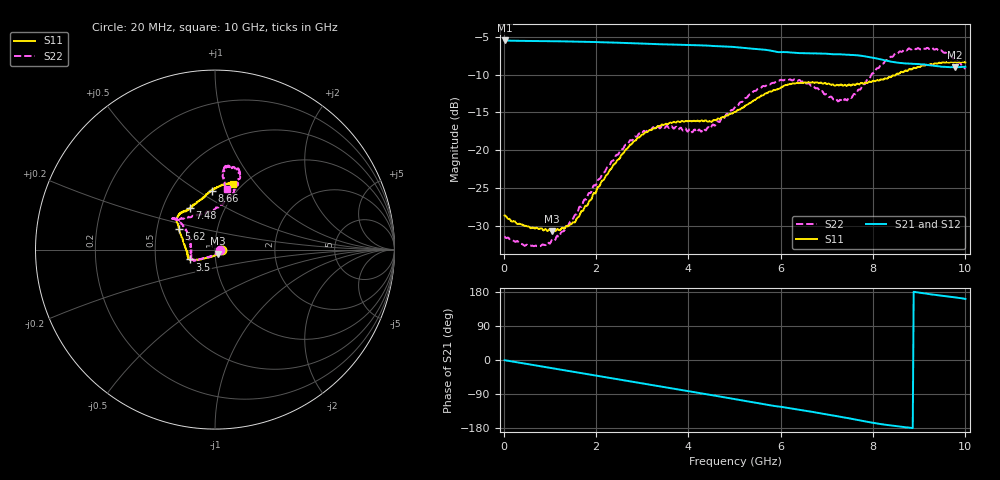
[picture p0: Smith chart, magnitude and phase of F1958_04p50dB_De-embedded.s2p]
! Integrated Device Technology
! Corporate Headquarters
! 6024 Silver Creek Valley Road
! San Jose, CA 95138  USA
! Phone:  1-408-284-8200
! Toll Free:  1-800-223-1366
! Webpage:  http://www.idt.com/
! Timing and RF Division
! 515 Groton Road, Suite 102
! Westford, MA 01886-6024
! Device:  F1958
! Description: 7-bit 0.25 dB Digital Step Attenuator
! Frequency:  0.001 -  6.000 GHz
! Package:  4x4 mm Thin QFN Plastic Package: 24 pin
! Ports:  2 RF, 12 DC
!  Pin  1  = D0
!  Pin  2  = VDD
!  Pin  3  = VMODE
!  Pin  4  = GND
!  Pin  5  = RF1  =  Port 1
!  Pin  6  = GND
!  Pin  7  = GND
!  Pin  8  = GND
!  Pin  9  = GND
!  Pin 10  = GND
!  Pin 11  = GND
!  Pin 12  = GND
!  Pin 13  = GND
!  Pin 14  = RF2  =  Port 2
!  Pin 15  = GND
!  Pin 16  = LE
!  Pin 17  = CLK
!  Pin 18  = DATA
!  Pin 19  = D6
!  Pin 20  = D5
!  Pin 21  = D4
!  Pin 22  = D3
!  Pin 23  = D2
!  Pin 24  = D1
! State:  18
! Atten State:  4.50 dB
! Voltage:  +3.30 Volts
! Current:  0.258 mA
! Data:  The device was measured on a F1958 evaluation board which has
!  individual transmission lines to the RF pins.  Data was collected
!  using a calibrated network analyzer.  The evaluation board was
!  de-embedded using Automatic Fixture Removal (AFR).
!  The reference plane is the edge of the package pin.
! Misc:
!  Action Tracker AT0419
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# GHz S dB R 50
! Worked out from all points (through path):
!   500 points, 20 MHz to 10 GHz, reference 50 ohm
!   highest |S21| = -5.51 dB at 20 MHz (marker M1); lowest = -9.0 dB at 9.78 GHz (marker M2)
!   group delay of S21, straight-line fit = 56.3 ps
!   lowest |S11| = -30.7 dB at 1.04 GHz (marker M3), VSWR 1.06, Z = 51.8 - j2.38 ohm
!   |S11| at or under -10 dB: start of sweep to 8.497 GHz
!   |S22| runs from -32.6 to -6.5 dB; largest |S21 - S12| = 0.0017
!   S11 on the Smith chart (normalised r, x): 20 MHz: 1.08, -0.00; 3.5 GHz: 0.75, -0.08; 5.62 GHz: 0.65, +0.16; 7.48 GHz: 0.68, +0.34; 8.66 GHz: 0.78, +0.57; 10 GHz: 0.91, +0.78
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0.02  -28.60 -3.4  -5.51 -0.6  -5.51 -0.5  -31.36 -4.3
0.56  -30.14 -21.0  -5.57 -11.6  -5.57 -11.6  -32.58 -29.7
1.04  -30.68 -51.6  -5.60 -21.4  -5.60 -21.4  -31.84 -69.3
1.42  -29.89 -86.6  -5.64 -29.3  -5.64 -29.3  -29.62 -104.0
1.7  -28.00 -107.4  -5.68 -34.9  -5.67 -34.9  -27.27 -122.2
2.6  -20.32 -145.9  -5.83 -53.5  -5.82 -53.5  -19.67 -148.8
2.96  -18.17 -152.6  -5.91 -61.0  -5.90 -61.0  -17.82 -151.4
3.36  -16.83 -156.6  -6.00 -69.1  -6.00 -69.2  -16.98 -155.4
3.5  -16.52 -158.6  -6.02 -72.0  -6.03 -72.1  -16.99 -159.3
4.32  -16.16 -170.8  -6.16 -88.9  -6.18 -88.9  -17.17 173.2
5.02  -14.94 166.9  -6.38 -103.6  -6.39 -103.6  -14.19 146.5
5.62  -12.74 150.4  -6.71 -116.2  -6.72 -116.2  -11.50 141.6
6.18  -11.27 141.6  -7.08 -126.9  -7.09 -126.9  -10.69 143.2
6.68  -11.02 134.4  -7.21 -136.7  -7.23 -136.6  -11.46 139.2
7.22  -11.35 126.5  -7.33 -148.2  -7.35 -148.0  -13.40 115.6
7.48  -11.31 121.3  -7.40 -153.9  -7.41 -153.8  -13.02 95.1
7.96  -11.00 109.9  -7.74 -165.0  -7.74 -165.0  -10.06 73.4
8.34  -10.35 100.7  -8.23 -172.1  -8.24 -172.1  -7.97 70.4
8.66  -9.68 93.1  -8.52 -176.6  -8.53 -176.6  -6.78 72.4
9.3  -8.66 80.0  -8.82 172.5  -8.83 172.5  -6.58 82.8
9.78  -8.31 75.6  -9.05 165.1  -9.07 165.2  -7.92 83.0
10  -8.41 74.5  -8.98 161.1  -9.01 161.2  -9.27 79.2
